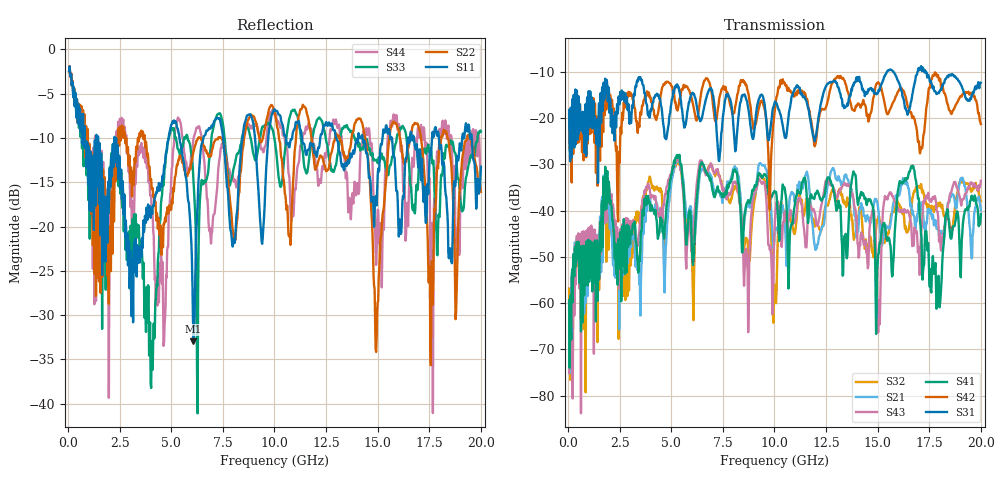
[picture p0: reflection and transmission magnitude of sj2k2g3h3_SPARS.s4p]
! FILE: E:\users\goganessyan\GBX_Backplane\FR408_backplane\1m_INBOUND_NEXT\sj2k2g3h3_SPARS.s4p
# MHZ S RI R 50.00
! FREQ  S11  S12  S13  S14
!  S21  S22  S23  S24
!  S31  S32  S33  S34
!  S41  S42  S43  S44
!  REAL  IMAG  REAL  IMAG  REAL  IMAG  REAL  IMAG
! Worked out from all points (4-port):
!   799 points, 50 MHz to 20 GHz, reference 50 ohm
!   strongest paths, dB at 50 MHz, 5.025 GHz, 10.03 GHz, 15.03 GHz, 20 GHz:
!     S31: -18.3, -16.0, -16.4, -14.4, -12.4
!     S42: -19.2, -13.3, -17.9, -12.3, -21.3
!     S41: -59.3, -32.1, -35.9, -49.5, -40.7
!     S43: -75.1, -31.6, -41.8, -66.3, -33.6
!     S21: -61.2, -33.2, -45.0, -39.7, -39.9
!     S32: -56.8, -32.6, -56.3, -41.7, -37.9
!   lowest |S11| = -32.9 dB at 6.075 GHz (marker M1), VSWR 1.05, Z = 52.3 + j0.297 ohm
!   |S11| at or under -10 dB: 2.251 GHz to 4.87 GHz (2.619 GHz wide, 73.6 % of centre); 5.396 GHz to 6.556 GHz (1.16 GHz wide, 19.4 % of centre); 17.97 GHz to 19.1 GHz (1.129 GHz wide, 6.09 % of centre)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
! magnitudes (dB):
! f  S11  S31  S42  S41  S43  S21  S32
! 50 MHz  -2.4  -18.3  -19.2  -59.3  -75.1  -61.2  -56.8
! 1.95 GHz  -14.9  -13.3  -13.7  -38.1  -38.4  -40.5  -48.4
! 6.075 GHz  -32.9  -14.8  -17.6  -50.4  -43.7  -45.2  -63.7
! 13.53 GHz  -13.0  -16.9  -14.1  -49.9  -34.6  -33.1  -37.2
! 15.05 GHz  -13.8  -13.9  -12.4  -49.3  -59.3  -40.6  -41.1
! 15.38 GHz  -9.0  -10.6  -17.8  -43.7  -37.2  -43.3  -45.9
! 20 GHz  -13.2  -12.4  -21.3  -40.7  -33.6  -39.9  -37.9
